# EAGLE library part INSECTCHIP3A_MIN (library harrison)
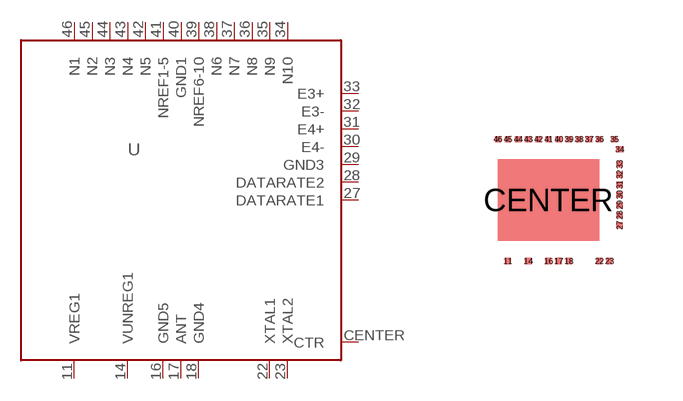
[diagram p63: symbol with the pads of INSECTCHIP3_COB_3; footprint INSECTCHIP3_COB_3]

Designator prefix U

## INSECTCHIP3A_MIN  [INSECTCHIP3_COB_3]
11  VREG1  pwr
14  VUNREG1  pwr
16  GND5  pwr
17  ANT  pas
18  GND4  pwr
22  XTAL1  pas
23  XTAL2  pas
27  DATARATE1  in
28  DATARATE2  in
29  GND3  pwr
30  E4-  in
31  E4+  in
32  E3-  in
33  E3+  in
34  N10  in
35  N9  in
36  N8  in
37  N7  in
38  N6  in
39  NREF6-10  in
40  GND1  pwr
41  NREF1-5  in
42  N5  in
43  N4  in
44  N3  in
45  N2  in
46  N1  in
CENTER  CTR  pwr

## Footprint INSECTCHIP3_COB_3 (pad centres in mm)
smd 0.152 x 0.152: 11 -1.016,-1.524; 14 -0.508,-1.524; 16 0,-1.524; 17 0.254,-1.524; 18 0.508,-1.524; 22 1.27,-1.524; 23 1.524,-1.524; 27 1.778,-0.635; 28 1.778,-0.381; 29 1.778,-0.127; 30 1.778,0.127; 31 1.778,0.381; 32 1.778,0.635; 33 1.778,0.889; 34 1.778,1.27; 35 1.651,1.524; 36 1.27,1.524; 37 1.016,1.524; 38 0.762,1.524; 39 0.508,1.524; 40 0.254,1.524; 41 0,1.524; 42 -0.254,1.524; 43 -0.508,1.524; 44 -0.762,1.524; 45 -1.016,1.524; 46 -1.27,1.524
smd 2.54 x 2.032: CENTER 0,0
